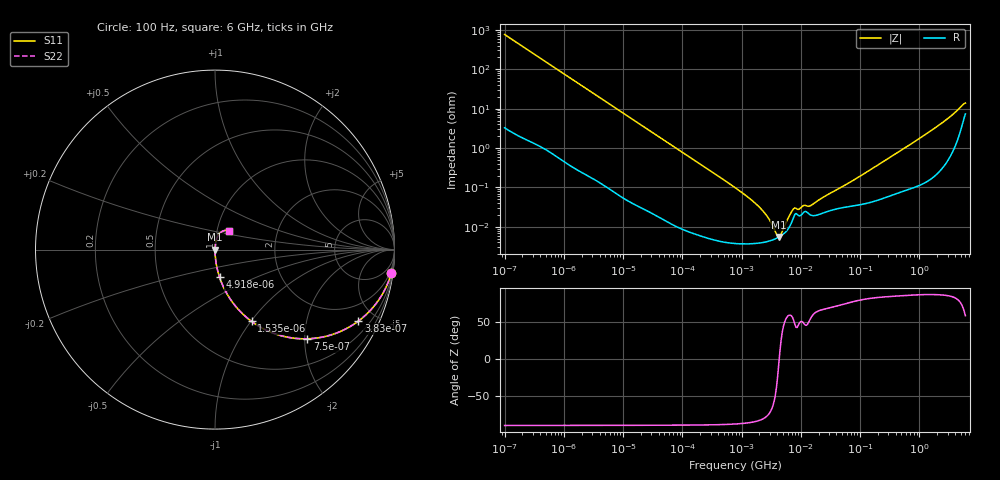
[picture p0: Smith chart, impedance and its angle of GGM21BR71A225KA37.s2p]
!Murata Part Number: GGM21BR71A225KA37
!These Parameters are Measured in Series Mode Connection
!Data Generated on Mar 13, 2026
!  o--ll--o
!Port1  Port2
!  o------o
!Operation Temp=25[degC], DC Bias Voltage=0[V]
!Freq. Start=100[Hz] Stop=6[GHz] 401[Steps]
# Hz S RI R 50
!Freq.(Hz) S11(Real) S11(Imag) S21(Real) S21(Imag) S12(Real) S12(Imag) S22(Real) S22(Imag)
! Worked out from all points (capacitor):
!   401 points, 100 Hz to 6 GHz, reference 50 ohm
!   read as one part in series: C = 2.08 uF near 109 Hz
!   lowest |Z| = 5.51 mohm at 4.246 MHz (marker M1)
!   series resonance near 4.323 MHz, so ESL is about 650 pH
!   S11 on the Smith chart (normalised r, x): 100 Hz: 1, -15; 383 Hz: 1.02, -4.01; 750 Hz: 1.01, -2.05; 1.535 kHz: 1.01, -1.01; 4.918 kHz: 1.00, -0.32; 6 GHz: 1.15, +0.24
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100  0.9827 -0.1283  0.0173 0.1283  0.0173 0.1283  0.9827 -0.1283
214  0.9266 -0.2584  0.0734 0.2584  0.0734 0.2584  0.9266 -0.2584
383  0.7995 -0.3976  0.2005 0.3976  0.2005 0.3976  0.7995 -0.3976
750  0.5134 -0.4969  0.4866 0.4969  0.4866 0.4969  0.5134 -0.4969
1535  0.2034 -0.3996  0.7966 0.3996  0.7966 0.3996  0.2034 -0.3996
2008  0.1306 -0.3339  0.8694 0.3339  0.8694 0.3339  0.1306 -0.3339
4918  0.0253 -0.1537  0.9747 0.1537  0.9747 0.1537  0.0253 -0.1537
12041  0.00462 -0.0644  0.9954 0.0644  0.9954 0.0644  0.00462 -0.0644
40335  0.000552 -0.0194  0.9994 0.0194  0.9994 0.0194  0.000552 -0.0194
774597  3.87e-05 -0.000992  1 0.000992  1 0.000992  3.87e-05 -0.000992
1983483  3.88e-05 -0.000317  1 0.000317  1 0.000317  3.88e-05 -0.000317
2594782  4.16e-05 -0.000197  1 0.000197  1 0.000197  4.16e-05 -0.000197
3394479  4.68e-05 -9.12e-05  1 9.12e-05  1 9.12e-05  4.68e-05 -9.12e-05
4246196  5.47e-05 -6.7e-06  0.9999 6.7e-06  0.9999 6.7e-06  5.47e-05 -6.7e-06
4856642  6.23e-05 4.48e-05  0.9999 -4.48e-05  0.9999 -4.48e-05  6.23e-05 4.48e-05
5311619  6.96e-05 8.07e-05  0.9999 -8.07e-05  0.9999 -8.07e-05  6.96e-05 8.07e-05
7599586  0.00018 0.000227  0.9998 -0.000227  0.9998 -0.000227  0.00018 0.000227
1.555665e7  0.000193 0.000309  0.9998 -0.000309  0.9998 -0.000309  0.000193 0.000309
3.124326e8  0.000634 0.00563  0.9994 -0.00563  0.9994 -0.00563  0.000634 0.00563
1.95892e9  0.00333 0.0344  0.9967 -0.0344  0.9967 -0.0344  0.00333 0.0344
4.009986e9  0.0168 0.0771  0.9832 -0.0771  0.9832 -0.0771  0.0168 0.0771
6e9  0.0793 0.1013  0.9207 -0.1013  0.9207 -0.1013  0.0793 0.1013
